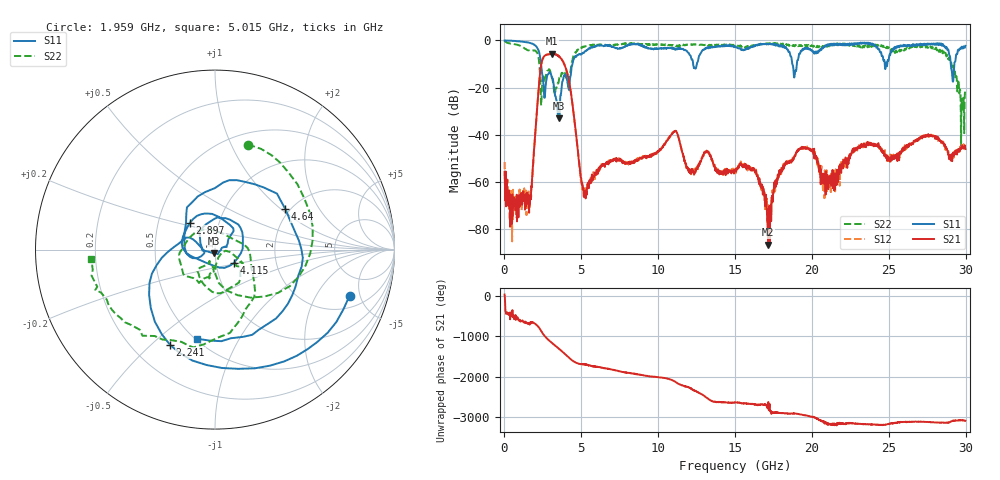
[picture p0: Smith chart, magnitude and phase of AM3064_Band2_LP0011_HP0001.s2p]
# Hz S DB R 50.0
!freq dBS11 angS11 dBS21 angS21 dBS12 angS12 dBS22 angS22
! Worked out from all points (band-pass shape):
!   1600 points, 10 MHz to 29.98 GHz, reference 50 ohm
!   highest |S21| = -5.68 dB at 3.084 GHz (marker M1); lowest = -86.5 dB at 17.16 GHz (marker M2)
!   |S21| within 3 dB of the highest: 2.444 GHz to 3.786 GHz (1.342 GHz wide, 43.1 % of centre)
!   lowest |S11| = -33.0 dB at 3.571 GHz (marker M3), VSWR 1.05, Z = 49.3 - j2.12 ohm
!   |S11| at or under -10 dB: 2.382 GHz to 4.421 GHz (2.039 GHz wide, 60 % of centre); 12.27 GHz to 12.51 GHz (238.3 MHz wide, 1.92 % of centre); 18.73 GHz to 19.02 GHz (294.2 MHz wide, 1.56 % of centre)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
!   |S22| runs from -45.0 to -0.2 dB; largest |S21 - S12| = 0.015
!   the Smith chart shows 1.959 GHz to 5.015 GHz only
!   S11 on the Smith chart (normalised r, x): 1.959 GHz: 2.87, -3.99; 2.241 GHz: 0.36, -0.58; 2.897 GHz: 0.73, +0.23; 4.115 GHz: 1.22, -0.18; 4.64 GHz: 1.89, +1.07; 5.015 GHz: 0.51, -0.68
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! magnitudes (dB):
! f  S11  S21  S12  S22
! 10 MHz  0.0  -55.7  -51.5  -0.2
! 441.1 MHz  -0.1  -68.3  -70.3  -1.4
! 1.584 GHz  -0.9  -67.8  -66.2  -4.3
! 1.959 GHz  -2.0  -43.4  -43.7  -4.2
! 2.241 GHz  -4.6  -19.2  -19.2  -8.4
! 2.897 GHz  -13.8  -5.9  -5.8  -12.2
! 3.084 GHz  -15.6  -5.7  -5.7  -15.8
! 3.571 GHz  -33.0  -6.8  -6.8  -15.7
! 4.115 GHz  -17.8  -14.7  -14.6  -18.3
! 4.64 GHz  -6.9  -38.8  -38.7  -5.2
! 5.015 GHz  -5.9  -60.2  -59.6  -3.2
! 10 GHz  -3.5  -47.2  -46.6  -1.8
! 15 GHz  -2.5  -55.3  -54.7  -1.8
! 16.32 GHz  -2.3  -55.5  -55.7  -2.0
! 17.16 GHz  -1.7  -86.5  -76.6  -1.4
! 18.19 GHz  -2.4  -53.6  -53.5  -1.9
! 19.99 GHz  -4.1  -46.6  -46.7  -2.0
! 20.83 GHz  -2.8  -60.0  -55.0  -2.4
! 25 GHz  -8.0  -49.6  -50.8  -2.9
! 28.56 GHz  -2.1  -43.4  -43.7  -4.6
! 29.18 GHz  -17.5  -48.1  -49.2  -10.2
! 29.98 GHz  -2.3  -46.0  -45.7  -21.7
